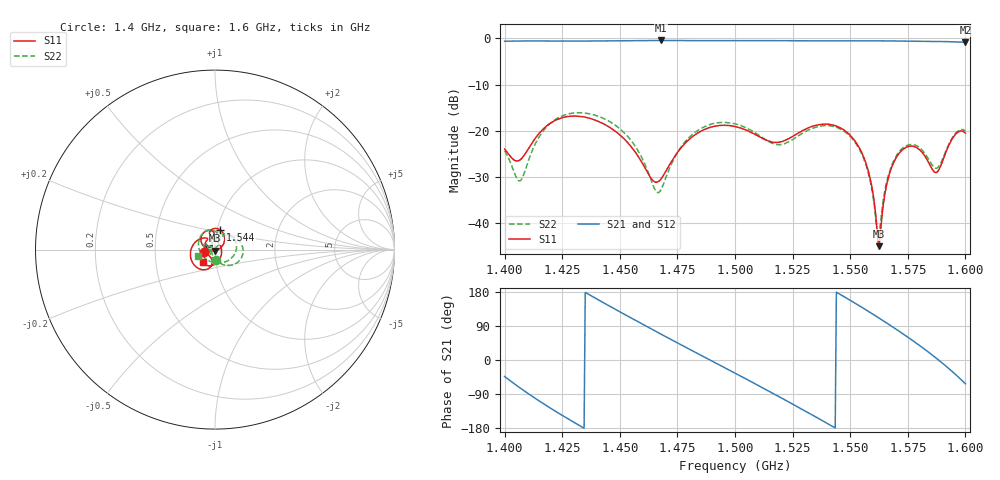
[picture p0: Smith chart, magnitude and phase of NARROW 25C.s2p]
!Agilent Technologies,E8364B,MY43040699,A.07.50.67
!Agilent E8364B: A.07.50.67
!Date: Wednesday, June 25, 2025 05:42:33
!Correction: S11(Full 2 Port(1,2))
!S21(Full 2 Port(1,2))
!S12(Full 2 Port(1,2))
!S22(Full 2 Port(1,2))
!S2P File: Measurements: S11, S21, S12, S22:
# Hz S  dB  R 50
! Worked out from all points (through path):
!   401 points, 1.4 GHz to 1.6 GHz, reference 50 ohm
!   highest |S21| = -0.46 dB at 1.468 GHz (marker M1); lowest = -0.9 dB at 1.6 GHz (marker M2)
!   lowest |S11| = -44.9 dB at 1.562 GHz (marker M3), VSWR 1.01, Z = 50.1 - j0.564 ohm
!   |S11| at or under -10 dB: start of sweep to end of sweep
!   |S22| runs from -42.6 to -16.1 dB; largest |S21 - S12| = 0.0013
!   S11 on the Smith chart (normalised r, x): 1.4 GHz: 0.88, -0.02; 1.544 GHz: 1.03, +0.23; 1.6 GHz: 0.87, -0.12
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1.4e9  -23.95 -167.5  -0.63 -43.4  -0.63 -43.4  -24.29 -83.0
1.407e9  -26.16 -121.3  -0.58 -75.0  -0.57 -75.0  -30.71 158.5
1.4145e9  -20.82 -102.8  -0.57 -106.0  -0.57 -106.0  -21.70 64.2
1.4245e9  -17.22 -128.1  -0.60 -144.2  -0.59 -144.2  -16.88 18.8
1.4335e9  -16.91 -161.3  -0.59 -176.5  -0.59 -176.5  -16.09 -9.9
1.4425e9  -18.36 163.0  -0.56 152.5  -0.55 152.5  -17.21 -34.9
1.452e9  -21.78 128.0  -0.51 120.5  -0.50 120.5  -20.45 -62.1
1.467e9  -30.86 147.8  -0.47 71.1  -0.47 71.1  -33.28 177.3
1.468e9  -30.33 154.3  -0.46 67.8  -0.46 67.8  -32.69 157.9
1.476e9  -24.01 163.8  -0.48 41.9  -0.48 42.0  -23.90 90.4
1.4845e9  -20.26 144.2  -0.51 14.7  -0.50 14.7  -19.68 58.0
1.5e9  -19.06 105.3  -0.52 -34.6  -0.52 -34.6  -18.46 1.7
1.517e9  -22.48 99.4  -0.50 -89.8  -0.50 -89.8  -22.83 -98.6
1.5335e9  -19.03 101.0  -0.55 -144.9  -0.55 -144.9  -19.47 144.1
1.5435e9  -18.87 75.5  -0.56 -179.3  -0.56 -179.3  -19.14 101.3
1.556e9  -25.85 30.2  -0.54 135.5  -0.54 135.5  -26.16 58.8
1.5625e9  -44.91 -82.2  -0.54 110.7  -0.55 110.7  -42.59 134.0
1.567e9  -29.36 -177.7  -0.57 93.0  -0.56 93.0  -28.90 179.1
1.576e9  -23.30 133.4  -0.62 56.1  -0.62 56.1  -22.97 156.3
1.586e9  -28.56 38.5  -0.66 11.3  -0.65 11.3  -27.68 162.5
1.5925e9  -23.46 -74.0  -0.73 -21.0  -0.72 -21.0  -23.23 -149.9
1.6e9  -20.50 -133.5  -0.85 -62.8  -0.85 -62.8  -20.00 -160.2
